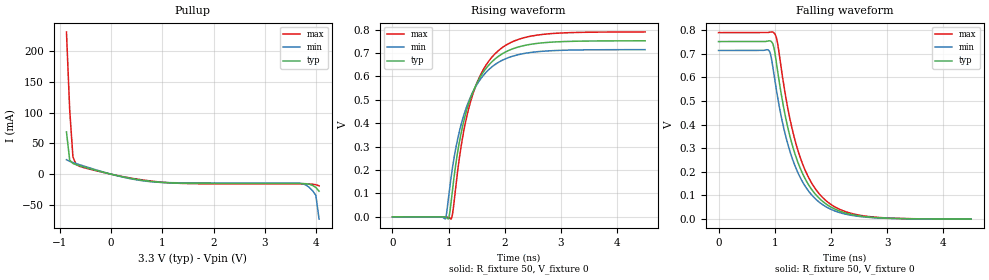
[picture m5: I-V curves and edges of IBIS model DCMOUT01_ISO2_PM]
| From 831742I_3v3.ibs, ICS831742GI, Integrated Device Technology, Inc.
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[Model]   DCMOUT01_ISO2_PM
Model_type   Open_source
Polarity   Non-Inverting
|   typ   min   max
C_comp   2pF   1.5pF   2.5pF
Vmeas = 0.37V
Rref = 50
Cref = 0
Vref = 0V
|   typ   min   max
[Voltage range]   3.3V   3.135V   3.465V
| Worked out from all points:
|   slope of the pullup table from 0 to 0.495 V, typ, clamps not added: 59.1 ohm
|   rising waveform, R_fixture 50, V_fixture 0: 20-80 % time 486ps typ, 490ps min, 483ps max; typ from 0 V to 0.752 V
|   falling waveform, R_fixture 50, V_fixture 0: 20-80 % time 521ps typ, 519ps min, 523ps max; typ from 0.752 V to 0 V
[Pullup]
|Voltage   I (typ)   I (min)   I (max)
|Note, modeling breaks down at 250mA and above.  This is well beyond the functional   |
|operating range of the device.  Should this scenario occur, catastrophic failure and   |
|possible damage to the device and/or board is of higher concern than the I-V curve   |
|behavior.  The IBIS checker will flag currents in excess of 10A with warnings.  Lines   |
|with currents in excess of 0.35 A have been commented out.  The points still remain|
|available to the user if the user desires to use them.   |
|-2.84000e+00   4.81596e+00   5.86293e+00   4.19710e+00
|-2.38000e+00   3.70245e+00   4.44558e+00   3.26690e+00
|-1.92000e+00   2.59033e+00   3.02976e+00   2.33731e+00
|-1.46000e+00   1.48086e+00   1.61455e+00   1.41033e+00
|-1.00000e+00   3.73332e-01   2.01387e-01   4.86599e-01
|-9.99000e-01   3.70928e-01   1.98320e-01   4.84593e-01
|-9.35793e-01   2.19003e-01   4.10084e-02   3.57880e-01
-872.6mV  68.77mA    23.56mA    231.2mA
-809.4mV  22.97mA    20.91mA    104.7mA
-746.2mV  17.41mA    19.03mA    27.98mA
-683mV    15.39mA    17.28mA    15.8mA
-493.3mV  10.78mA    12.23mA    9.831mA
138.7mV   -2.666mA   -2.993mA   -2.446mA
770.8mV   -11.6mA    -12.19mA   -11.05mA
1.529V    -14.71mA   -14.1mA    -15.24mA
3.742V    -15.2mA    -15.52mA   -15.88mA
3.868V    -16.34mA   -21.63mA   -15.99mA
3.994V    -21.49mA   -34.23mA   -17.07mA
4.058V    -27.61mA   -72.86mA   -18.93mA
| 4.12076e+00   -5.61169e-02   -4.54233e-01   -2.37305e-02
| 4.18397e+00   -2.95373e-01   -9.54703e-01   -4.47327e-02
| 4.24717e+00   -6.86892e-01   -1.45540e+00   -1.85181e-01
| 4.31038e+00   -1.07878e+00   -1.95626e+00   -5.10850e-01
| 4.37359e+00   -1.47095e+00   -2.45725e+00   -8.36947e-01
| 4.43679e+00   -1.86334e+00   -2.95832e+00   -1.16339e+00
| 4.50000e+00   -2.25590e+00   -3.45946e+00   -1.49014e+00
| 4.50100e+00   -2.26212e+00   -3.46739e+00   -1.49531e+00
| 4.92080e+00   -4.87188e+00   -6.79644e+00   -3.66992e+00
| 5.34060e+00   -7.48321e+00   -1.01253e+01   -5.84808e+00
| 5.76040e+00   -1.00947e+01   -1.34536e+01   -8.02733e+00
| 6.18020e+00   -1.27060e+01   -1.67815e+01   -1.02069e+01
| 6.60000e+00   -1.53173e+01   -2.01093e+01   -1.23867e+01
[Ramp]
|   typ   min   max
dV/dt_r   0.456/0.485n   0.434/0.489n   0.479/0.481n
dV/dt_f   0.453/0.521n   0.43/0.518n   0.475/0.523n
R_load =   50.0000
[Rising Waveform]
R_fixture = 50
V_fixture = 0   | VCC_typ
V_fixture_max = 0   | VCC_max
V_fixture_min = 0   | VCC_min
C_fixture = 0.0p
| Time   typ   min   max
0s        1.469nV    331.2pV    95.28nV
936.9ps   -1.485mV   -9.435mV   134.1uV
1ns       -5.913mV   87.18mV    -2.851mV
1.05ns    76.48mV    180.2mV    -7.094mV
1.203ns   335mV      377.1mV    272.1mV
1.401ns   514.3mV    518.8mV    501.6mV
1.635ns   624.8mV    609.4mV    636.8mV
1.946ns   695.6mV    668mV      721.8mV
2.68ns    743.8mV    707.7mV    779.7mV
4.495ns   752.2mV    714.4mV    790mV
[Falling Waveform]
R_fixture = 50
V_fixture = 0   | VCC_typ
V_fixture_max = 0   | VCC_max
V_fixture_min = 0   | VCC_min
C_fixture = 0.0p
| Time   typ   min   max
0s        752.2mV    714.4mV    790.1mV
882.9ps   754.6mV    716.5mV    790.7mV
932.4ps   753.5mV    692.3mV    792.8mV
1.004ns   703.3mV    584.8mV    783.9mV
1.203ns   420.6mV    344.6mV    509.1mV
1.428ns   230.8mV    188.7mV    279.7mV
1.667ns   122.6mV    99.91mV    148.8mV
1.968ns   55.24mV    44.84mV    67.28mV
2.689ns   8.285mV    6.644mV    10.19mV
4.495ns   71.73uV    55.7uV     90.84uV
